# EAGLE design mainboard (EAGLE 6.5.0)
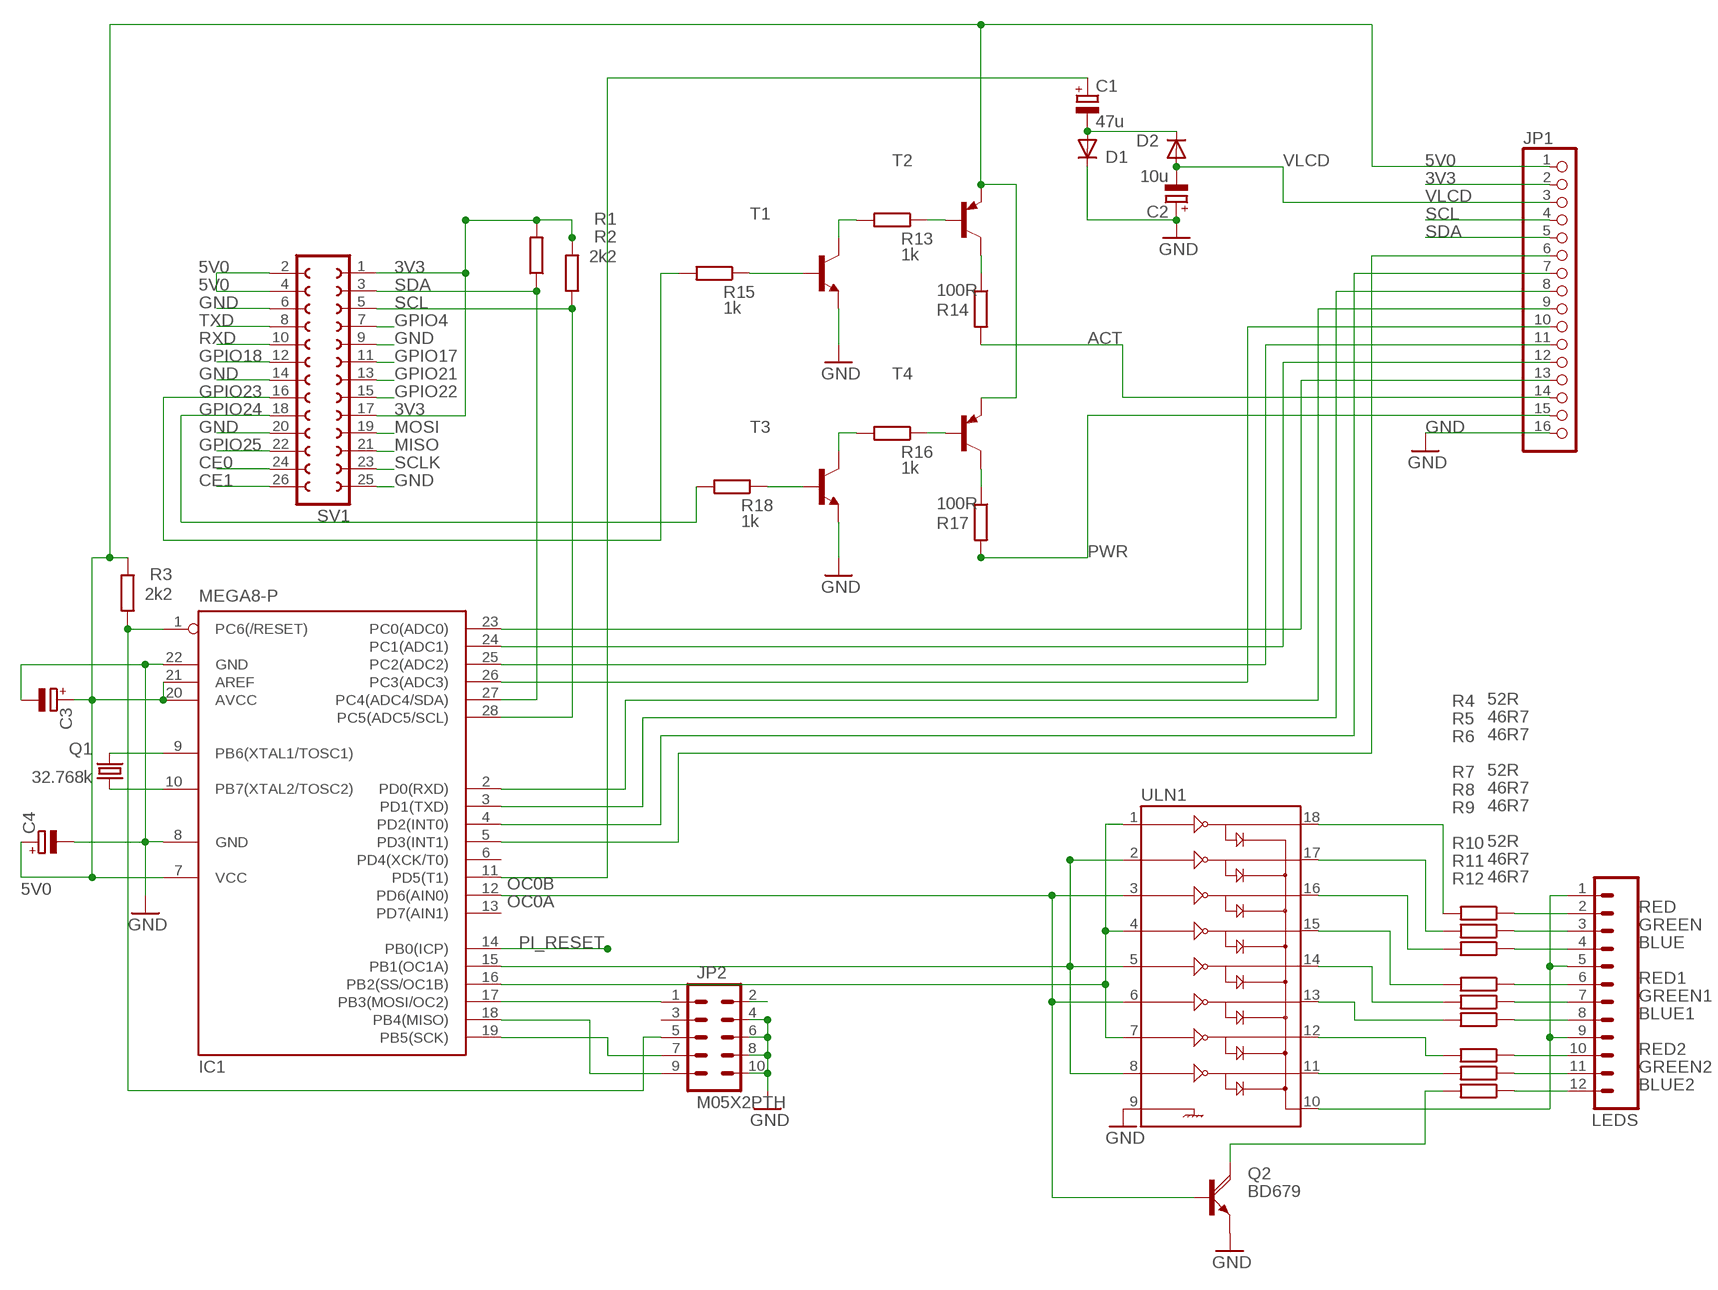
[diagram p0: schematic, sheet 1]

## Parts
C1  47u  CPOL-EUE2.5-6  [E2,5-6]
C2  10u  CPOL-EUE2.5-6  [E2,5-6]
C3  CPOL-EUE2.5-6  [E2,5-6]
C4  CPOL-EUE2.5-6  [E2,5-6]
D1  1N4148DO35-7  [DO35-7]
D2  1N4148DO35-7  [DO35-7]
IC1  MEGA8-P  [DIL28-3]
JP1  PINHD-1X16  [1X16]
JP2  M05X2PTH  [AVR_ICSP]
LEDS  M12LONGPADS  [1X12_LONGPADS]
Q1  32.768k  CRYSTALTC26V  [TC26V]
Q2  BD679  [TO126AV]
R1  2k2  R-EU_0204/5  [0204/5]
R2  2k2  R-EU_0204/7  [0204/7]
R3  2k2  R-EU_0207/10  [0207/10]
R4  52R  R-EU_0204/7  [0204/7]
R5  46R7  R-EU_0204/7  [0204/7]
R6  46R7  R-EU_0204/7  [0204/7]
R7  52R  R-EU_0204/7  [0204/7]
R8  46R7  R-EU_0204/7  [0204/7]
R9  46R7  R-EU_0204/7  [0204/7]
R10  52R  R-EU_0204/7  [0204/7]
R11  46R7  R-EU_0204/7  [0204/7]
R12  46R7  R-EU_0204/7  [0204/7]
R13  1k  R-EU_0204/2V  [0204V]
R14  100R  R-EU_0207/15  [0207/15]
R15  1k  R-EU_0204/7  [0204/7]
R16  1k  R-EU_0204/7  [0204/7]
R17  100R  R-EU_0207/15  [0207/15]
R18  1k  R-EU_0207/10  [0207/10]
SV1  FE13-2  [FE13-2]
T1  -NPN-TO92-EBC  [TO92-EBC]
T2  BC450-PNP-TO92-EBC  [TO92-EBC]
T3  -NPN-TO92-EBC  [TO92-EBC]
T4  BC450-PNP-TO92-EBC  [TO92-EBC]
ULN1  ULN2803DIP  [DIL18]

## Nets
3V3: JP1.2 R1.2 R2.2 SV1.1 SV1.17
5V0: C3.+ C4.+ IC1.7(VCC) IC1.20(AVCC) IC1.21(AREF) JP1.1 JP2.2 LEDS.1 LEDS.5 LEDS.9 R3.2 SV1.2 SV1.4 T2.E T4.E ULN1.10
A: IC1.23(PC0(ADC0)) JP1.13
ACT: JP1.14 R14.2
B: IC1.24(PC1(ADC1)) JP1.12
BLUE: LEDS.4 R6.1
BLUE1: LEDS.8 R9.1
BLUE2: LEDS.12 R12.1
C: IC1.25(PC2(ADC2)) JP1.11
CE0: SV1.24
CE1: SV1.26
D: IC1.26(PC3(ADC3)) JP1.10
E: IC1.2(PD0(RXD)) JP1.9
F: IC1.3(PD1(TXD)) JP1.8
G: IC1.4(PD2(INT0)) JP1.7
GND: C2.+ C3.- C4.- D1.C IC1.8(GND) IC1.22(GND) JP1.16 JP2.4 JP2.6 JP2.8 JP2.10 Q2.E SV1.6 SV1.9 SV1.14 SV1.20 SV1.25 T1.E T3.E ULN1.9
GPIO4: SV1.7
GPIO17: SV1.11
GPIO18: SV1.12
GPIO21: SV1.13
GPIO22: SV1.15
GPIO23: R15.2 SV1.16
GPIO24: R18.2 SV1.18
GPIO25: SV1.22
GREEN: LEDS.3 R5.1
GREEN1: LEDS.7 R8.1
GREEN2: LEDS.11 R11.1
H: IC1.5(PD3(INT1)) JP1.6
MISO: SV1.21
MOSI: SV1.19
N$1: IC1.9(PB6(XTAL1/TOSC1)) Q1.2
N$2: C1.- D1.A D2.C
N$3: IC1.10(PB7(XTAL2/TOSC2)) Q1.1
N$11: IC1.15(PB1(OC1A)) ULN1.2 ULN1.5 ULN1.8
N$13: IC1.12(PD6(AIN0)) Q2.B ULN1.3 ULN1.6
N$14: R4.2 ULN1.18
N$15: IC1.1(PC6(/RESET)) JP2.5 R3.1
N$16: R5.2 ULN1.17
N$17: R6.2 ULN1.16
N$18: R7.2 ULN1.15
N$19: R8.2 ULN1.14
N$20: IC1.17(PB3(MOSI/OC2)) JP2.1
N$21: IC1.18(PB4(MISO)) JP2.9
N$22: IC1.19(PB5(SCK)) JP2.7
N$23: R9.2 ULN1.13
N$24: R10.2 ULN1.12
N$25: R11.2 ULN1.11
N$26: Q2.C R12.2
N$30: R14.1 T2.C
N$31: R13.1 T2.B
N$32: R13.2 T1.C
N$33: R15.1 T1.B
N$35: R17.1 T4.C
N$36: R16.1 T4.B
N$37: R16.2 T3.C
N$38: R18.1 T3.B
OC0A: C1.+ IC1.11(PD5(T1))
OC0B: IC1.16(PB2(SS/OC1B)) ULN1.1 ULN1.4 ULN1.7
PI_RESET: IC1.14(PB0(ICP))
PWR: JP1.15 R17.2
RED: LEDS.2 R4.1
RED1: LEDS.6 R7.1
RED2: LEDS.10 R10.1
RXD: SV1.10
SCL: IC1.28(PC5(ADC5/SCL)) JP1.4 R1.1 SV1.5
SCLK: SV1.23
SDA: IC1.27(PC4(ADC4/SDA)) JP1.5 R2.1 SV1.3
TXD: SV1.8
VLCD: C2.- D2.A JP1.3
Unconnected: IC1.6(PD4(XCK/T0)) IC1.13(PD7(AIN1)) JP2.3

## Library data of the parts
C1-C4 = rcl:CPOL-EU: POLARIZED CAPACITOR, European symbol
D1 D2 = diode:1N4148: DIODE
IC1 = atmel:MEGA8-P: MICROCONTROLLER 8 Kbytes FLASH, 1 kbytes SRAM, 512 bytes EEPROM, USART, 4-channel 10 bit ADC, 2-channel 8 bit ADC Pin compatible with Atmega48, ATMega88, ATMega168 Source: avr.lbr; OC_FARNELL: unknown; OC_NEWARK: unknown
JP1 = pinhead:PINHD-1X16: PIN HEADER
JP2 = SparkFun:M05X2: Header 5x2 Standard 10-pin dual row 0.1" header. Commonly used with AVR-ISP. Use with Spark Fun Electronics SKU: PRT-00778
LEDS = SparkFun:M12: Header 12 Standard 12-pin 0.1" header. Use with straight break away headers (SKU : PRT-00116), right angle break away headers (PRT-00553), swiss pins (PRT-00743), machine pins (PRT-00117), and female headers (PRT-00115).
Q1 = crystal:CRYSTAL: CRYSTAL; OC_FARNELL: unknown; OC_NEWARK: unknown
Q2 = transistor-power:BD679: NPN DARLINGTON TRANSISTOR
R1-R18 = rcl:R-EU_: RESISTOR, European symbol
SV1 = con-lsta:FE13-2: FEMALE HEADER; OC_FARNELL: unknown; OC_NEWARK: unknown
T1 T3 = transistor:*-NPN-: NPN Transistror BF959 corrected 2008.03.06
T2 T4 = transistor:*-PNP-: PNP Transistror
ULN1 = SparkFun:ULN2803: Darlington Driver ULN2803 Darlington array. 500mA max per channel, 8-channel package. Spark Fun Electronics SKU : COM-00312

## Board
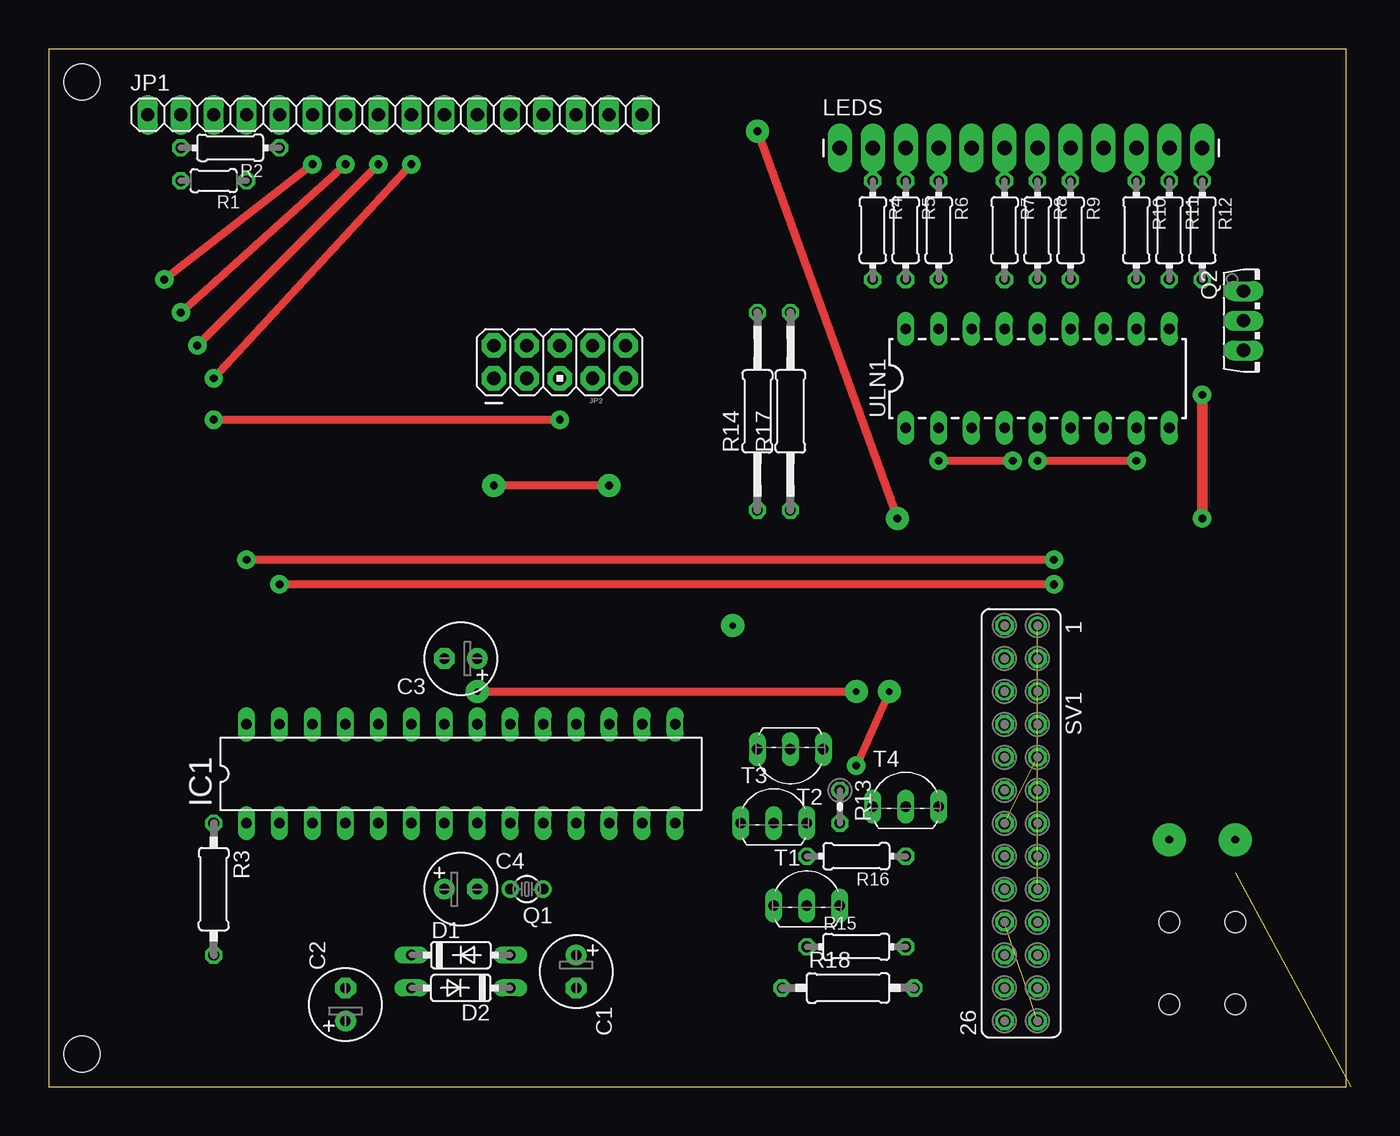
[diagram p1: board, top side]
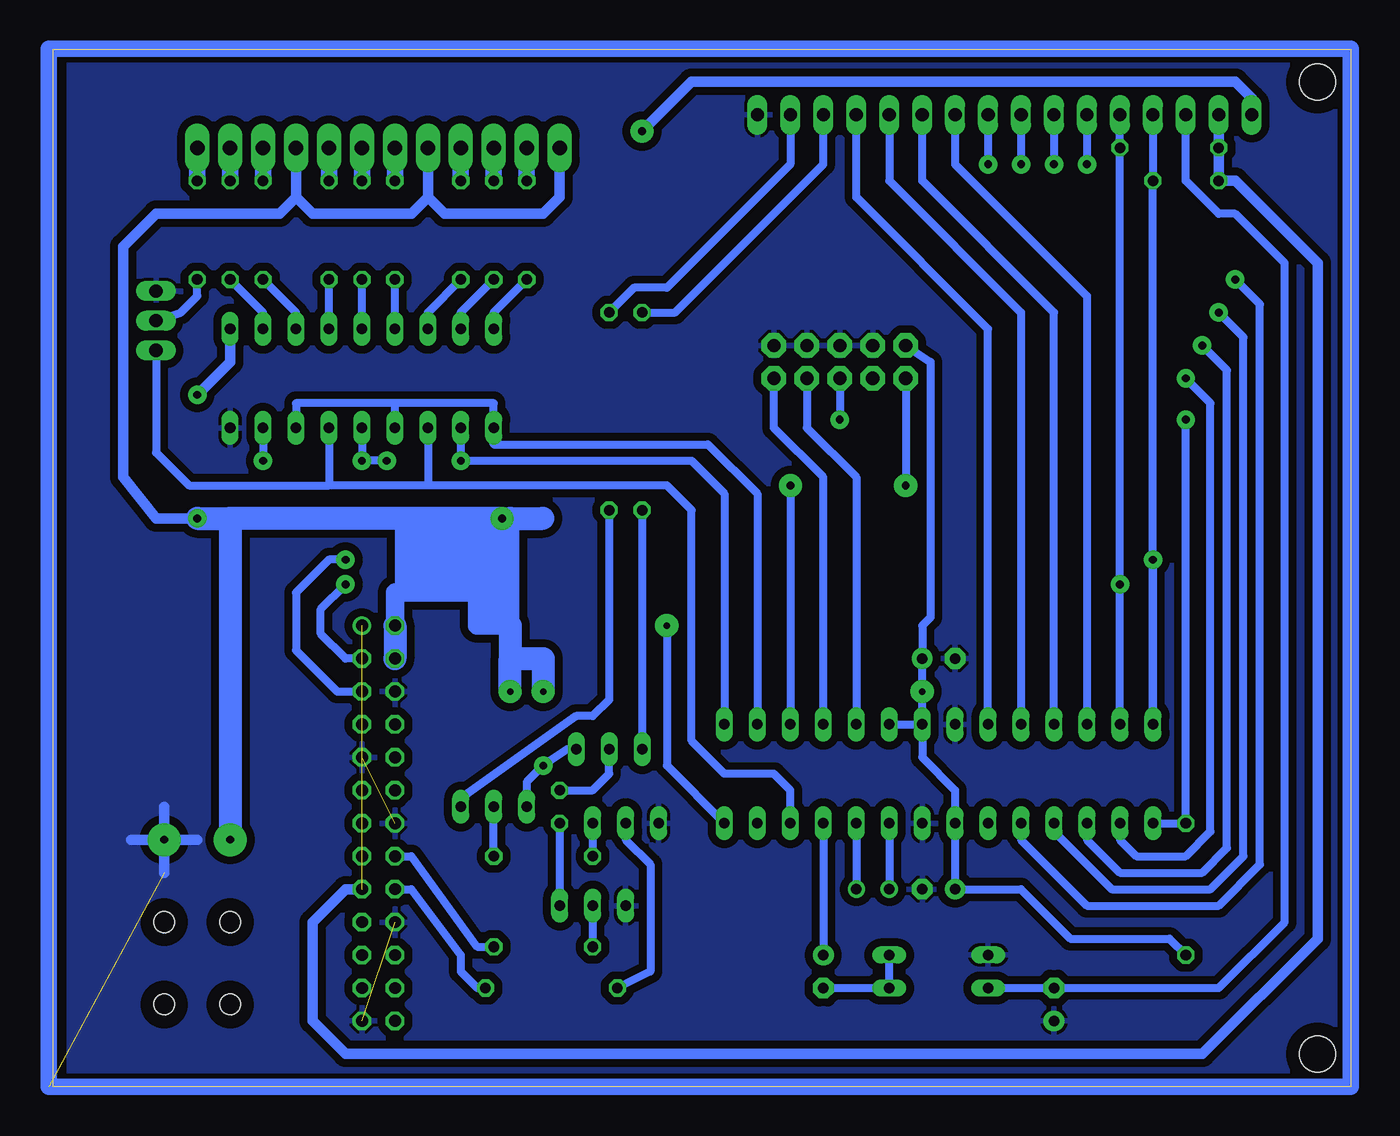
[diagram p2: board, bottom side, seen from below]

Size 100 x 80 mm. Coordinates in mm from the lower left corner, seen from the top.
Outline: 0,0 100,0 100,80 0,80 0,0
Copper layers (1*16): Top 0.035mm / dielectric 1.5mm / Bottom 0.035mm
Design rules "default": minimum track width 10mil, minimum drill 24mil, track to track 8mil, track to pad 8mil, pad to pad 8mil, via to via 8mil, smd to smd 8mil, copper to edge 40mil, drill to drill 8mil, minimum pad ring 10mil, minimum via ring 8mil, stop-mask expansion 4mil, vias tented up to drill 0mil, thermal gap 10mil
Holes 2.8 mm at 2.54,2.54 2.54,77.47
Holes 1.6 mm at 86.36,12.7 91.44,12.7 91.44,6.35 86.36,6.35
tRestrict: area 80,21.6 to 99.1,29.2

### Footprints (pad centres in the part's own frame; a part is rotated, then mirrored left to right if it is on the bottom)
E2,5-6 = drill 0.813 pad 1.6: + -1.27,0 | drill 0.813 pad 1.6 octagon: - 1.27,0
DO35-7 = drill 0.813 long: A 3.81,0; C -3.81,0
DIL28-3 = drill 0.813 long: 1 -16.51,-3.81; 2 -13.97,-3.81; 3 -11.43,-3.81; 4 -8.89,-3.81; 5 -6.35,-3.81; 6 -3.81,-3.81; 7 -1.27,-3.81; 8 1.27,-3.81; 9 3.81,-3.81; 10 6.35,-3.81; 11 8.89,-3.81; 12 11.43,-3.81; 13 13.97,-3.81; 14 16.51,-3.81; 15 16.51,3.81; 16 13.97,3.81; 17 11.43,3.81; 18 8.89,3.81; 19 6.35,3.81; 20 3.81,3.81; 21 1.27,3.81; 22 -1.27,3.81; 23 -3.81,3.81; 24 -6.35,3.81; 25 -8.89,3.81; 26 -11.43,3.81; 27 -13.97,3.81; 28 -16.51,3.81
1X16 = drill 1.016 long: 1 -19.05,0; 2 -16.51,0; 3 -13.97,0; 4 -11.43,0; 5 -8.89,0; 6 -6.35,0; 7 -3.81,0; 8 -1.27,0; 9 1.27,0; 10 3.81,0; 11 6.35,0; 12 8.89,0; 13 11.43,0; 14 13.97,0; 15 16.51,0; 16 19.05,0
AVR_ICSP = drill 1.016 pad 1.88 octagon: 1 -1.27,5.08; 2 1.27,5.08; 3 -1.27,2.54; 4 1.27,2.54; 5 -1.27,0; 6 1.27,0; 7 -1.27,-2.54; 8 1.27,-2.54; 9 -1.27,-5.08; 10 1.27,-5.08
1X12_LONGPADS = drill 1.118 pad 1.88 long: 1 0,0; 2 2.54,0; 3 5.08,0; 4 7.62,0; 5 10.16,0; 6 12.7,0; 7 15.24,0; 8 17.78,0; 9 20.32,0; 10 22.86,0; 11 25.4,0; 12 27.94,0
TC26V = drill 0.813: 1 -1.27,0; 2 1.27,0
TO126AV = drill 1.016 long: B 2.286,-1.27; C 0,-1.27; E -2.286,-1.27
0204/5 = drill 0.813 octagon: 1 -2.54,0; 2 2.54,0
0204/7 = drill 0.813 octagon: 1 -3.81,0; 2 3.81,0
0207/10 = drill 0.813 octagon: 1 -5.08,0; 2 5.08,0
0204V = drill 0.813 octagon: 1 -1.27,0; 2 1.27,0
0207/15 = drill 0.813 octagon: 1 -7.62,0; 2 7.62,0
FE13-2 = drill 0.914: 1 -15.24,1.27 | drill 0.914 octagon: 2 -15.24,-1.27; 3 -12.7,1.27; 4 -12.7,-1.27; 5 -10.16,1.27; 6 -10.16,-1.27; 7 -7.62,1.27; 8 -7.62,-1.27; 9 -5.08,1.27; 10 -5.08,-1.27; 11 -2.54,1.27; 12 -2.54,-1.27; 13 0,1.27; 14 0,-1.27; 15 2.54,1.27; 16 2.54,-1.27; 17 5.08,1.27; 18 5.08,-1.27; 19 7.62,1.27; 20 7.62,-1.27; 21 10.16,1.27; 22 10.16,-1.27; 23 12.7,1.27; 24 12.7,-1.27; 25 15.24,1.27; 26 15.24,-1.27
TO92-EBC = drill 0.813 long: B 0,-1.27; C 2.54,-1.27; E -2.54,-1.27
DIL18 = drill 0.813 long: 1 -10.16,-3.81; 2 -7.62,-3.81; 3 -5.08,-3.81; 4 -2.54,-3.81; 5 0,-3.81; 6 2.54,-3.81; 7 5.08,-3.81; 8 7.62,-3.81; 9 10.16,-3.81; 10 10.16,3.81; 11 7.62,3.81; 12 5.08,3.81; 13 2.54,3.81; 14 0,3.81; 15 -2.54,3.81; 16 -5.08,3.81; 17 -7.62,3.81; 18 -10.16,3.81

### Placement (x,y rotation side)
C1  40.64,8.89 270 top
C2  22.86,6.35 90 top
C3  31.75,33.02 180 top
C4  31.75,15.24 0 top
D1  31.75,10.16 0 top
D2  31.75,7.62 180 top
IC1  31.75,24.13 0 top
JP1  26.67,74.93 0 top
JP2  39.37,55.88 90 top
LEDS  60.96,72.39 0 top
Q1  36.83,15.24 180 top
Q2  93.34,59.05 270 top
R1  12.7,69.85 180 top
R2  13.97,72.39 180 top
R3  12.7,15.24 270 top
R4  63.5,66.04 270 top
R5  66.04,66.04 270 top
R6  68.58,66.04 270 top
R7  73.66,66.04 270 top
R8  76.2,66.04 270 top
R9  78.74,66.04 270 top
R10  83.82,66.04 270 top
R11  86.36,66.04 270 top
R12  88.9,66.04 270 top
R13  60.96,21.59 270 top
R14  54.61,52.07 90 top
R15  62.23,10.79 0 top
R16  62.23,17.78 180 top
R17  57.15,52.07 90 top
R18  61.59,7.62 0 top
SV1  74.93,20.32 270 top
T1  58.42,15.24 0 top
T2  57.15,24.77 180 top
T3  55.88,21.59 0 top
T4  66.04,22.86 0 top
ULN1  76.2,54.61 0 top

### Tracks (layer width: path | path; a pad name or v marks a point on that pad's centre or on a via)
3V3  (1 unrouted)
  Bottom 0.813: SV1.17 77.47,15.24 80.01,12.7 80.01,5.08 77.47,2.54 11.43,2.54 2.54,11.43 2.54,63.5 8.89,69.85 R1.2 R2.2 JP1.2
5V0  (via drill 0.5 pad 1.78, 0.6 pad 1.42, 0.6 pad 1.78, 0.6 pad 2.54)
  Top 0.61: v54.61,73.66 v65.41,43.81 | v33.02,30.48 v62.23,30.48 | v64.77,30.48 v62.23,24.77
  Top 0.813: v88.9,53.34 v88.9,43.81
  Bottom 0.61: JP2.2 32.38,55.88 32.38,36.2 33.02,35.56 C3.+ v33.02,30.48 IC1.21 | T4.E 63.5,23.5 v62.23,24.77 60.33,26.04 T2.E | IC1.21 33.02,25.4 30.48,22.86 IC1.7 C4.+ 25.4,15.24 21.59,11.43 13.97,11.43 R3.2 | IC1.20 IC1.21
  Bottom 0.813: v88.9,43.81 92.08,43.81 94.61,46.99 94.61,64.77 92.08,67.31 82.55,67.31 81.28,68.58 | LEDS.9 81.28,68.58 | 81.28,68.58 80.01,67.31 72.39,67.31 71.12,68.58 | LEDS.5 71.12,68.58 | 71.12,68.58 69.85,67.31 62.23,67.31 60.96,68.58 LEDS.1 | ULN1.10 86.36,55.88 v88.9,53.34 | v54.61,73.66 50.8,77.47 8.89,77.47 7.62,76.2 JP1.1
  Bottom 1.27: 73.66,35.82 SV1.2
  Bottom 1.422: 64.77,43.81 64.77,35.56 67.31,35.56 67.31,38.1 73.66,38.1 SV1.4
  Bottom 1.778: 86.36,43.81 v65.41,43.81 64.77,43.81 62.27,43.81 | 86.36,43.81 v86.36,19.05 | v88.9,43.81 86.36,43.81 | 64.77,35.56 64.77,33.02 | v64.77,30.48 64.77,33.02 | 64.77,33.02 62.23,33.02 v62.23,30.48 | SV1.2 SV1.4
A
  Bottom 0.61: IC1.23 27.94,58.42 38.1,68.58 JP1.13
ACT
  Bottom 0.61: R14.2 52.07,59.69 40.64,71.12 JP1.14
B
  Bottom 0.61: JP1.12 35.56,69.85 25.4,59.69 IC1.24
BLUE
  Bottom 1.27: LEDS.4 R6.1
BLUE1
  Bottom 1.27: LEDS.8 R9.1
BLUE2
  Bottom 1.27: LEDS.12 R12.1
C
  Bottom 0.61: IC1.25 22.86,59.69 33.02,69.85 JP1.11
D
  Bottom 0.61: JP1.10 30.48,71.12 20.32,60.96 IC1.26
E  (via drill 0.6, 0.6 pad 1.42)
  Top 0.61: v12.7,54.61 v27.94,71.12
  Bottom 0.61: IC1.2 17.78,19.05 16.51,17.78 12.7,17.78 10.79,19.68 10.79,52.7 v12.7,54.61 | JP1.9 v27.94,71.12
F  (via drill 0.6, 0.6 pad 1.42)
  Top 0.61: v11.43,57.15 v25.4,71.12
  Bottom 0.61: IC1.3 20.32,19.05 17.78,16.51 11.43,16.51 9.53,18.41 9.53,55.24 v11.43,57.15 | JP1.8 v25.4,71.12
G  (via drill 0.6, 0.6 pad 1.42)
  Top 0.61: v10.16,59.69 v22.86,71.12
  Bottom 0.61: IC1.4 22.86,19.68 18.41,15.24 10.79,15.24 8.26,17.78 8.26,57.78 v10.16,59.69 | JP1.7 v22.86,71.12
GND  (3 unrouted)
  Bottom 0.813: 93.98,19.05 88.9,19.05 | 91.44,21.59 91.44,16.51
  Bottom 1.27: 0,80.01 100.33,80.01 100.33,0 0,0 0,80.01
  pour Bottom (isolate 0.61): 0,80.01 100.33,80.01 100.33,0 0,0
GPIO23
  Bottom 0.61: SV1.16 72.39,17.78 67.31,10.79 R15.2
GPIO24
  Bottom 0.61: SV1.18 72.39,15.24 68.58,10.16 68.58,8.89 67.31,7.62 R18.2
GREEN
  Bottom 1.27: LEDS.3 R5.1
GREEN1
  Bottom 1.27: LEDS.7 R8.1
GREEN2
  Bottom 1.27: LEDS.11 R11.1
H  (via drill 0.6, 0.6 pad 1.42)
  Top 0.61: v8.89,62.23 v20.32,71.12
  Bottom 0.61: IC1.5 25.4,19.05 20.32,13.97 10.16,13.97 6.99,17.14 6.99,60.33 v8.89,62.23 | JP1.6 v20.32,71.12
N$1
  Bottom 0.61: IC1.9 Q1.2
N$2
  Bottom 0.61: C1.- D2.C D1.A
N$3
  Bottom 0.61: IC1.10 Q1.1
N$4  (via drill 0.6 pad 2.54)
  other vias: 91.44,19.05
N$11  (via drill 0.6, 0.6 pad 1.42)
  Top 0.61: v68.58,48.26 v74.3,48.26 | v76.2,48.26 v83.82,48.26
  Bottom 0.61: IC1.15 48.26,45.72 50.8,48.26 v68.58,48.26 ULN1.2 | ULN1.5 v76.2,48.26 v74.3,48.26 | ULN1.8 v83.82,48.26
N$13
  Bottom 0.61: IC1.12 43.18,22.86 44.45,24.13 48.26,24.13 50.8,26.67 50.8,44.45 52.7,46.35 71.12,46.35 | ULN1.3 71.12,46.35 | 71.12,46.35 78.74,46.35 | ULN1.6 78.74,46.35 | Q2.B 92.08,48.9 89.53,46.35 78.74,46.35
N$14
  Bottom 0.61: ULN1.18 66.04,59.69 R4.2
N$15  (via drill 0.6, 0.6 pad 1.42)
  Top 0.61: v12.7,51.44 v39.37,51.44
  Bottom 0.61: IC1.1 R3.1 v12.7,51.44 | JP2.5 v39.37,51.44
N$16
  Bottom 0.61: ULN1.17 68.58,59.69 R5.2
N$17
  Bottom 0.61: R6.2 71.12,59.69 ULN1.16
N$18
  Bottom 0.61: ULN1.15 R7.2
N$19
  Bottom 0.61: ULN1.14 R8.2
N$20  (via drill 0.6 pad 1.78)
  Top 0.61: v43.18,46.35 v34.29,46.35
  Bottom 0.61: JP2.1 v34.29,46.35 | v43.18,46.35 IC1.17
N$21
  Bottom 0.61: IC1.18 40.64,46.99 44.45,50.8 JP2.9
N$22
  Bottom 0.61: JP2.7 41.91,50.8 38.1,46.99 IC1.19
N$23
  Bottom 0.61: ULN1.13 R9.2
N$24
  Bottom 0.61: ULN1.12 81.28,59.69 R10.2
N$25
  Bottom 0.61: ULN1.11 83.82,59.69 R11.2
N$26
  Bottom 0.61: Q2.C 90.17,59.69 88.9,60.96 R12.2
N$30
  Bottom 0.61: R14.1 T2.C
N$31
  Bottom 0.61: R13.1 58.42,22.86 57.15,24.13 T2.B
N$32
  Bottom 0.61: R13.2 T1.C
N$33
  Bottom 0.61: T1.B R15.1
N$35
  Bottom 0.61: R17.1 57.15,29.84 58.42,28.57 59.69,28.57 68.58,22.23 T4.C
N$36
  Bottom 0.61: R16.1 T4.B
N$37
  Bottom 0.61: T3.C R16.2
N$38
  Bottom 0.61: T3.B 55.88,19.05 53.98,17.14 53.98,8.89 R18.1
OC0A
  Bottom 0.61: IC1.11 C1.+
OC0B
  Bottom 0.61: IC1.16 45.72,45.72 49.53,49.53 66.04,49.53 ULN1.1 66.04,52.7 73.66,52.7 | ULN1.4 73.66,52.7 | 73.66,52.7 81.28,52.7 ULN1.7
PI_RESET  (via drill 0.5 pad 1.78)
  Bottom 0.61: v52.7,35.56 52.7,24.77 IC1.14
PWR
  Bottom 0.61: JP1.15 43.18,71.12 52.7,61.59 55.24,61.59 R17.2
RED
  Bottom 1.27: R4.1 LEDS.2
RED1
  Bottom 1.27: LEDS.6 R7.1
RED2
  Bottom 1.27: LEDS.10 R10.1
SCL  (via drill 0.6 pad 1.42)
  Top 0.61: v15.24,40.64 v77.47,40.64
  Bottom 0.61: JP1.4 R1.1 IC1.28 v15.24,40.64 | v77.47,40.64 78.74,40.64 81.28,38.1 81.28,33.66 78.11,30.48 SV1.5
SDA  (via drill 0.6, 0.6 pad 1.42)
  Top 0.61: v77.47,38.73 v17.78,38.73
  Bottom 0.61: IC1.27 v17.78,38.73 R2.1 JP1.5 | SV1.3 77.47,33.02 79.38,34.92 79.38,36.83 v77.47,38.73
VLCD
  Bottom 0.61: D2.A C2.- 10.16,7.62 5.08,12.7 5.08,63.5 8.89,67.31 10.16,67.31 12.7,69.85 JP1.3
(copper drawn outside any net)
  shapes: Bottom area x2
